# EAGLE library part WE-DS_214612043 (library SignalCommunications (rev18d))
WE-DS D-SUB-Filter Connectors Bent 90° Characteristics Standard type filtered with 1000 pF High attenuation of more than 40 dB @ 180 MHz Choice of earthing metal sheet or high speed earthing clip Rated voltage: 100 VDC Rated current @ 20 ºC: 5 A Withstand voltage: 250 VRMS Insulation resistance: min. 1000 MΩ Operating temperature: –55 ºC to +125 ºC Applications Filtering of interfaces External connection to -printer -sensor -display Details see: http://katalog.we-online.de/en/pbs/Filter_abgewinkelt Created on 2015-05-04 2015 (C) Wurth Elektronik
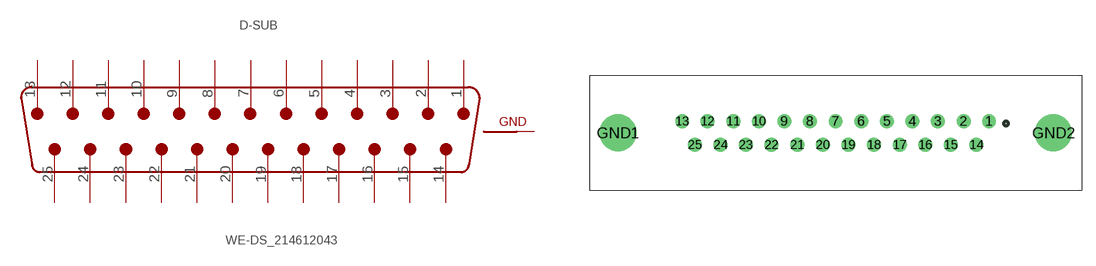
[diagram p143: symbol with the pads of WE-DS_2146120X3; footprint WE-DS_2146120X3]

Designator prefix D-SUB

## WE-DS_214612043 (WE-NUMBER: 514612043/25Pins_female)  [WE-DS_2146120X3]
1  13  pas
2  12  pas
3  11  pas
4  10  pas
5  9  pas
6  8  pas
7  7  pas
8  6  pas
9  5  pas
10  4  pas
11  3  pas
12  2  pas
13  1  pas
14  25  pas
15  24  pas
16  23  pas
17  22  pas
18  21  pas
19  20  pas
20  19  pas
21  18  pas
22  17  pas
23  16  pas
24  15  pas
25  14  pas
GND1  GND  pwr
GND2  GND  pwr

## Footprint WE-DS_2146120X3 (pad centres in mm)
drill 1: 1 16.56,1.27; 2 13.82,1.27; 3 11.05,1.27; 4 8.28,1.27; 5 5.54,1.27; 6 2.77,1.27; 7 0,1.27; 8 -2.77,1.27; 9 -5.54,1.27; 10 -8.28,1.27; 11 -11.05,1.27; 12 -13.82,1.27; 13 -16.56,1.27; 14 15.19,-1.27; 15 12.42,-1.27; 16 9.68,-1.27; 17 6.91,-1.27; 18 4.14,-1.27; 19 1.38,-1.27; 20 -1.38,-1.27; 21 -4.14,-1.27; 22 -6.91,-1.27; 23 -9.68,-1.27; 24 -12.42,-1.27; 25 -15.19,-1.27
drill 3: GND1 -23.5,0; GND2 23.5,0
